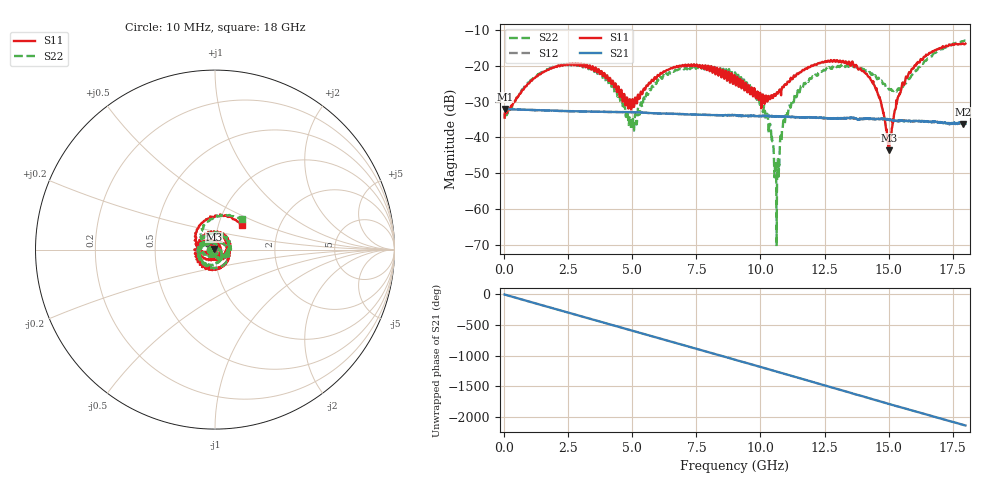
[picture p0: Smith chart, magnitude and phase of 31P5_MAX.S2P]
!Agilent Technologies,E5071C,MY46316741,A.11.02
!Date: Tue Sep 22 10:36:05 2020
!Data & Calibration Information:
!Freq	S11:SOLT4(ON)	S21:SOLT4(ON)	S12:SOLT4(ON)	S22:SOLT4(ON)
!PortZ  Port1:50+j0  Port2:50+j0
!Above PortZ is port z conversion or system Z0 setting when saving the data.
!When reading, reference impedance value at option line is always used.
# Hz S dB R 50
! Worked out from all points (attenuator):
!   1561 points, 10 MHz to 18 GHz, reference 50 ohm
!   highest |S21| = -32.03 dB at 21.53 MHz (marker M1); lowest = -36.2 dB at 17.91 GHz (marker M2)
!   lowest |S11| = -43.5 dB at 15.01 GHz (marker M3), VSWR 1.01, Z = 49.4 + j0.283 ohm
!   |S11| at or under -10 dB: start of sweep to end of sweep
!   |S22| runs from -70.3 to -12.9 dB; largest |S21 - S12| = 0.00072
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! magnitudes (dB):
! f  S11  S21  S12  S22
! 10 MHz  -34.5  -32.1  -32.0  -33.4
! 21.53 MHz  -33.1  -32.0  -32.1  -34.0
! 1.382 GHz  -22.4  -32.4  -32.4  -22.2
! 3.02 GHz  -19.6  -32.7  -32.7  -19.6
! 4.081 GHz  -24.1  -32.9  -32.9  -25.3
! 5.003 GHz  -29.3  -32.9  -33.0  -34.3
! 6.007 GHz  -22.6  -33.3  -33.3  -23.9
! 7.46 GHz  -20.1  -33.6  -33.6  -20.6
! 9.005 GHz  -23.4  -33.7  -33.9  -21.9
! 10.09 GHz  -28.0  -34.0  -34.0  -32.8
! 10.42 GHz  -28.2  -34.1  -34.0  -40.0
! 10.63 GHz  -27.5  -34.0  -34.1  -70.3
! 10.95 GHz  -25.3  -34.2  -34.3  -35.9
! 12.01 GHz  -20.0  -34.4  -34.4  -23.1
! 14.08 GHz  -22.0  -34.8  -34.8  -21.4
! 14.61 GHz  -28.4  -34.9  -34.9  -23.3
! 15 GHz  -43.4  -35.1  -35.0  -26.5
! 15.01 GHz  -43.5  -35.1  -35.1  -26.6
! 15.37 GHz  -28.7  -35.3  -35.6  -26.4
! 15.86 GHz  -21.9  -35.5  -35.4  -23.3
! 17.91 GHz  -13.9  -36.2  -36.2  -13.2
! 18 GHz  -13.8  -36.1  -36.1  -12.9
